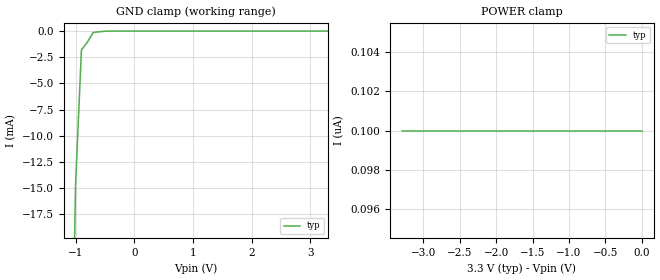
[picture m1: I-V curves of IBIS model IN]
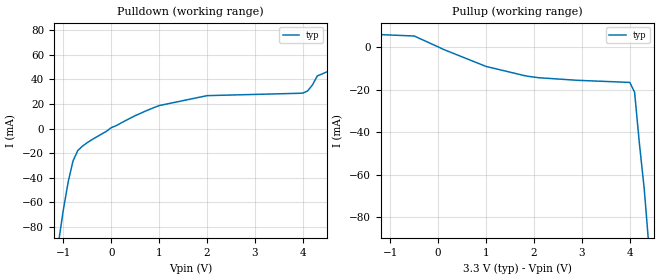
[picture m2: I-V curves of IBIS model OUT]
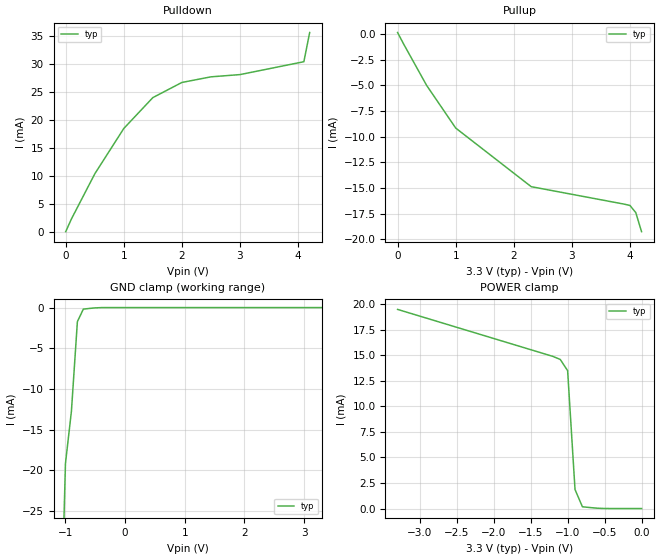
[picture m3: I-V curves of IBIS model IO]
|   Texas Instruments Incorporated
|   Bus Interface Products
|   IBIS Model for TL16C752BPT
|   48 pin TQFP Package
[IBIS Ver]   2.1
[Comment char]   |_char
[File name]   c752bpt.ibs
[File Rev]   1.0
[Date]   04Sep01
[Source]   File originated at Texas Instruments Incorporated.
   Data Transmission Products Group. All data based on
   Bench Measurements.
[Notes]   File created by Clarence Lewis
[Disclaimer]
(C) Copyright Texas Instruments Incorporated 2001
   All rights reserved
  Texas Instruments Incorporated hereby grants the user of this IBIS
model a non-exclusive, nontransferable license to use this IBIS model
under the following terms.  Before using this IBIS model, the user
should read this license.  If the user does not accept these terms,
the IBIS model should be returned to Texas Instruments within 30 days.
  The user is granted this license only to use the IBIS model and
is not granted rights to sell, load, rent, lease or license the IBIS
model in whole or in part, or in modified form to anyone other than
user.  User may modify the IBIS model to suit its specific applications
but rights to derivative works and such modifications shall belong to
Texas Instruments.
  This IBIS model is provided on an "AS IS" basis and Texas Instruments
makes absolutely no warranty with respect to the information contained
herein.  TEXAS INSTRUMENTS DISCLAIMS AND CUSTOMER WAIVES ALL WARRANTIES,
EXPRESS OR IMPLIED, INCLUDING WARRANTIES OF MERCHANTABILITY OR FITNESS
FOR A PARTICULAR PURPOSE. The entire risk as to quality and performance
is with the Customer. ACCORDINGLY, IN NO EVENT SHALL THE COMPANY BE LIABLE
FOR ANY DAMAGES, WHETHER IN CONTRACT OR TORT,INCLUDING ANY LOST PROFITS
OR OTHER INCIDENTAL, CONSEQUENTIAL, EXEMPLARY, OR PUNITIVE DAMAGES ARISING
OUT OF THE USE OR APPLICATION OF THE IBIS model provided in this package.
Further, Texas Instruments reserves the right to discontinue or make changes
without notice to any product herein to improve reliability, function, or
design. Texas Instruments does not convey any license under patent rights
or any other intellectual property rights, including those of third parties.
Contact Texas Instruments at ATTN:BUS INTERFACE
Clarence Lewis  8505 Forest Lane, M/S 8761, Dallas, TX 75243-4136
IBIS Open Forum disclaims all warranties. See DISCLAIM.TXT
in vhdl.org:/pub/IBIS/models for the full disclaimer.
[Copyright]   Copyright 2001, Texas Instruments, All Rights Reserved
[Component]   TL16C752BPT
[Manufacturer]  Texas Instruments Incorporated
[Package]
|   typ   min   max
R_pkg   0.068   0.063   0.071
L_pkg   3.205nH   2.995nH   3.507nH
C_pkg   0.574pF   0.500pF   0.629pF
[Pin]   signal_name   model_name   R_pin   L_pin   C_pin
1   D5   IO   0.070   3.018n   0.535p
2   D6   IO   0.069   3.040n   0.545p
3   D7   IO   0.067   3.272n   0.618p
4   RXB   IN   0.067   3.336n   0.623p
5   RXA   IN   0.064   3.373n   0.628p
6   TXRDYB#   OUT   0.063   3.412n   0.607p
7   TXA   OUT   0.063   3.473n   0.576p
8   TXB   OUT   0.066   3.338n   0.560p
9   OPB#   OUT   0.067   3.283n   0.616p
10   CSA#   IN   0.068   3.232n   0.614p
11   CSB#   IN   0.068   2.995n   0.543p
12   NC   NC
13   XTAL1   IN   0.070   3.010n   0.535p
14   XTAL2   OUT   0.071   3.019n   0.536p
15   IOW#   IN   0.070   3.045n   0.507p
16   CDB#   IN   0.068   3.391n   0.576p
17   GND   GND   0.066   3.425n   0.629p
18   RXRDYB#   OUT   0.064   3.507n   0.576p
19   IOR#   IN   0.066   3.392n   0.565p
20   DSRB#   IN   0.066   3.283n   0.617p
21   RIB#   IN   0.067   3.267n   0.616p
22   RTSB#   OUT   0.067   3.245n   0.615p
23   CTSB#   IN   0.069   3.029n   0.545p
24   NC   NC
25   NC   NC
26   A2   IN   0.070   3.006n   0.535p
27   A1   IN   0.069   3.010n   0.543p
28   A0   IN   0.069   3.230n   0.613p
29   INTB   OUT   0.067   3.234n   0.612p
30   INTA   OUT   0.064   3.301n   0.559p
31   RXRDYA#   OUT   0.066   3.360n   0.562p
32   OPA#   OUT   0.068   3.309n   0.619p
33   RTSA#   OUT   0.068   3.257n   0.616p
34   DTRA#   OUT   0.069   3.029n   0.547p
35   DTRB#   OUT   0.070   3.007n   0.537p
36   RESET   IN   0.070   2.995n   0.535p
37   NC   NC
38   CTSA#   IN   0.070   3.007n   0.534p
39   DSRA#   IN   0.069   3.018n   0.544p
40   CDA#   IN   0.067   3.216n   0.613p
41   RIA#   IN   0.067   3.255n   0.614p
42   VCC   POWER   0.066   3.337n   0.560p
43   TXRDYA#   OUT   0.063   3.323n   0.561p
44   D0   IO   0.066   3.294n   0.618p
45   D1   IO   0.067   3.235n   0.613p
46   D2   IO   0.069   3.036n   0.506p
47   D3   IO   0.070   3.033n   0.500p
48   D4   IO   0.070   3.018n   0.525p
| Models and submodels in the file (3): IN (Input), OUT (Output), IO (I/O)
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|   Input  MODEL
[Model]   IN
Model_type   Input
|Signals   RXA, RXB, CSA#, CSB#, XTAL1, IOW#, IOR#, A2, A1, A0, RESET,
|   CTSA#, DSRA#, CDA#, RIA#, CTSB#, DSRB#, CDB#, RIB#
Vinh = 2.0
Vinl = 0.8
|   typ   min   max
C_comp   5.4pF   NA   NA
|   typ   min   max
[Temperature Range]   25.0   NA   NA
[Voltage range]   3.3V   3.0V   3.6V
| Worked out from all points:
|   GND clamp passes 1 mA (typ) near -0.79 V on its own axis
[Power_clamp]
| Note that the POWER_clamp voltage table is referenced to Vcc
| and is calculated using Vtable = Vcc - Voutput.
|   Voltage   I(typ)   I(min)   I(max)
-3.3V     100nA      NA         NA
-3.2V     100nA      NA         NA
-100mV    100nA      NA         NA
0V        100nA      NA         NA
[GND_clamp]
|   Voltage   I(typ)   I(min)   I(max)
-3.3V     -602mA     NA         NA
-1.1V     -46.2mA    NA         NA
-1V       -14.6mA    NA         NA
-900mV    -1.796mA   NA         NA
-800mV    -1.073mA   NA         NA
-700mV    -136.6uA   NA         NA
-400mV    -900nA     NA         NA
3.3V      100nA      NA         NA
|   Output  MODEL
[Model]   OUT
Model_type   Output
| Signals   TXA, TXB, XTAL2, TXRDYA#, TXRDYB#, RXRDYA#, RXRDYB#, INTA, INTB,
|   RTSA#, DTRA#, RTSB#, DTRB#, OPA#, OPB#
| variable   typ   min   max
C_comp   10.0pF   NA   NA
|   typ   min   max
[Temperature Range]   25.0   NA   NA
[Voltage range]   3.3V   3.0V   3.6V
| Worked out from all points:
|   slope of the pulldown table from 0 to 0.495 V, typ, clamps not added: 51 ohm
|   slope of the pullup table from 0 to 0.495 V, typ, clamps not added: 106 ohm
[Pulldown]
|   Voltage   I(typ)   I(min)   I(max)
-3.3V     -733mA     NA         NA
-1.1V     -92.5mA    NA         NA
-900mV    -43.5mA    NA         NA
-800mV    -26.5mA    NA         NA
-700mV    -18mA      NA         NA
0V        700uA      NA         NA
1V        18.7mA     NA         NA
2V        26.8mA     NA         NA
4V        28.9mA     NA         NA
4.1V      30.7mA     NA         NA
4.3V      42.9mA     NA         NA
6.6V      82.5mA     NA         NA
[Pullup]
| Note that the[Pullup]voltage table is referenced to Vcc
| and is calculated using Vtable = Vcc - Voutput.
|   Voltage   I(typ)   I(min)   I(max)
-3.3V     7.8mA      NA         NA
-500mV    5.2mA      NA         NA
100mV     -1mA       NA         NA
1V        -9.1mA     NA         NA
1.8V      -13.4mA    NA         NA
2.9V      -15.6mA    NA         NA
4V        -16.6mA    NA         NA
4.1V      -21.2mA    NA         NA
4.2V      -45.2mA    NA         NA
4.3V      -66.3mA    NA         NA
4.4V      -94mA      NA         NA
6.6V      -731.6mA   NA         NA
[Ramp]
|   typ   min   max
dV/dt_r   1.98/5.6ns   NA   NA
dV/dt_f   1.98/4.5ns   NA   NA
|   I/O  MODEL
[Model]   IO
Model_type   I/O
|Signals   D0, D1, D2, D3, D4, D5, D6, D7
Vinh = 2.0
Vinl = 0.8
|   typ   min   max
C_comp   12.4pF   NA   NA
|   typ   min   max
[Temperature Range]   25.0   NA   NA
[Voltage range]   3.3V   3.0V   3.6V
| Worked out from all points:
|   slope of the pulldown table from 0 to 0.495 V, typ, clamps not added: 48.5 ohm
|   slope of the pullup table from 0 to 0.495 V, typ, clamps not added: 97.1 ohm
|   GND clamp passes 1 mA (typ) near -0.75 V on its own axis
|   POWER clamp passes 1 mA (typ) near -0.85 V on its own axis
[Power_clamp]   | Output tri-stated
| Note that the POWER_clamp voltage table is referenced to Vcc
| and is calculated using Vtable = Vcc - Voutput.
|   Voltage   I(typ)   I(min)   I(max)
-3.3V     19.5mA     NA         NA
-1.2V     14.9mA     NA         NA
-1.1V     14.6mA     NA         NA
-1V       13.5mA     NA         NA
-900mV    1.86mA     NA         NA
-800mV    170.4uA    NA         NA
-700mV    98.3uA     NA         NA
-600mV    31.5uA     NA         NA
-500mV    2.7uA      NA         NA
-400mV    200nA      NA         NA
-300mV    100nA      NA         NA
0V        100nA      NA         NA
[GND_clamp]   | Output tri-stated
|   Voltage   I(typ)   I(min)   I(max)
-3.3V     -607.6mA   NA         NA
-1.1V     -46.2mA    NA         NA
-1V       -19.15mA   NA         NA
-900mV    -12.73mA   NA         NA
-800mV    -1.726mA   NA         NA
-700mV    -187.8uA   NA         NA
-400mV    -3.1uA     NA         NA
3.3V      100nA      NA         NA
[Pullup]
| Note that the[Pullup]voltage table is referenced to Vcc
| and is calculated using Vtable = Vcc - Voutput.
|   Voltage   I(typ)   I(min)   I(max)
0V        130uA      NA         NA
100mV     -950uA     NA         NA
500mV     -5.02mA    NA         NA
1V        -9.17mA    NA         NA
2.3V      -14.88mA   NA         NA
3.9V      -16.58mA   NA         NA
4V        -16.71mA   NA         NA
4.1V      -17.4mA    NA         NA
4.2V      -19.26mA   NA         NA
[Pulldown]
|   Voltage   I(typ)   I(min)   I(max)
0V        100uA      NA         NA
100mV     2.4mA      NA         NA
500mV     10.4mA     NA         NA
1V        18.5mA     NA         NA
1.5V      24mA       NA         NA
2V        26.7mA     NA         NA
2.5V      27.7mA     NA         NA
3V        28.1mA     NA         NA
4.1V      30.4mA     NA         NA
4.2V      35.6mA     NA         NA
[Ramp]
|   typ   min   max
dV/dt_r   1.98/5.9ns   NA   NA
dV/dt_f   1.98/4.9ns   NA   NA
